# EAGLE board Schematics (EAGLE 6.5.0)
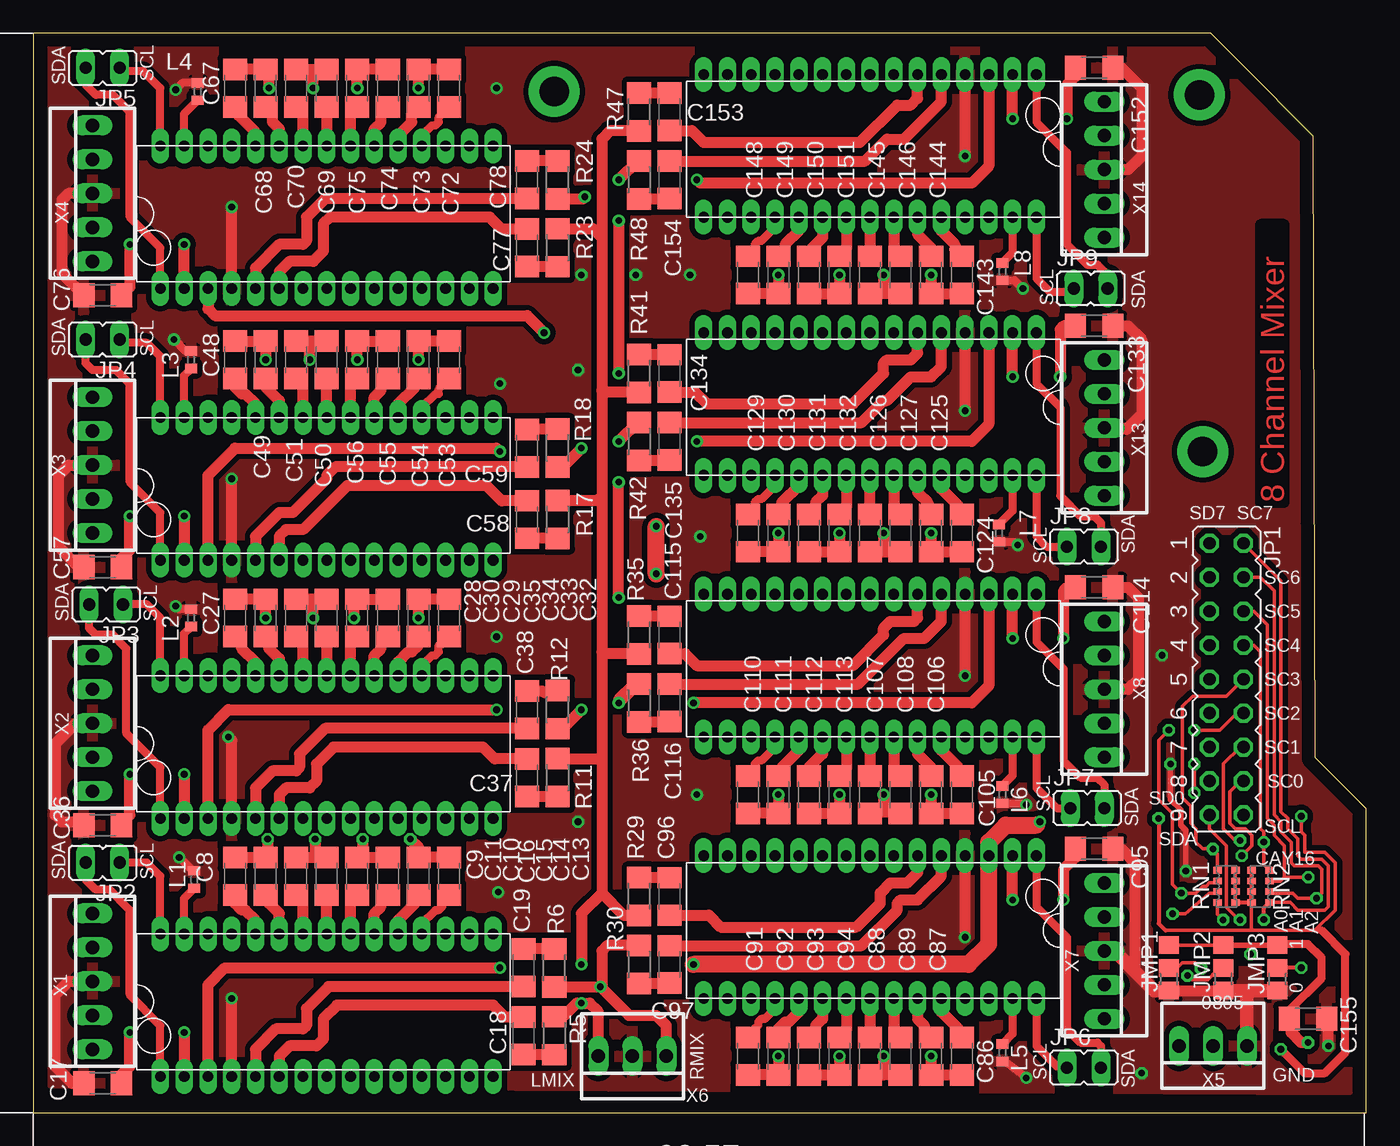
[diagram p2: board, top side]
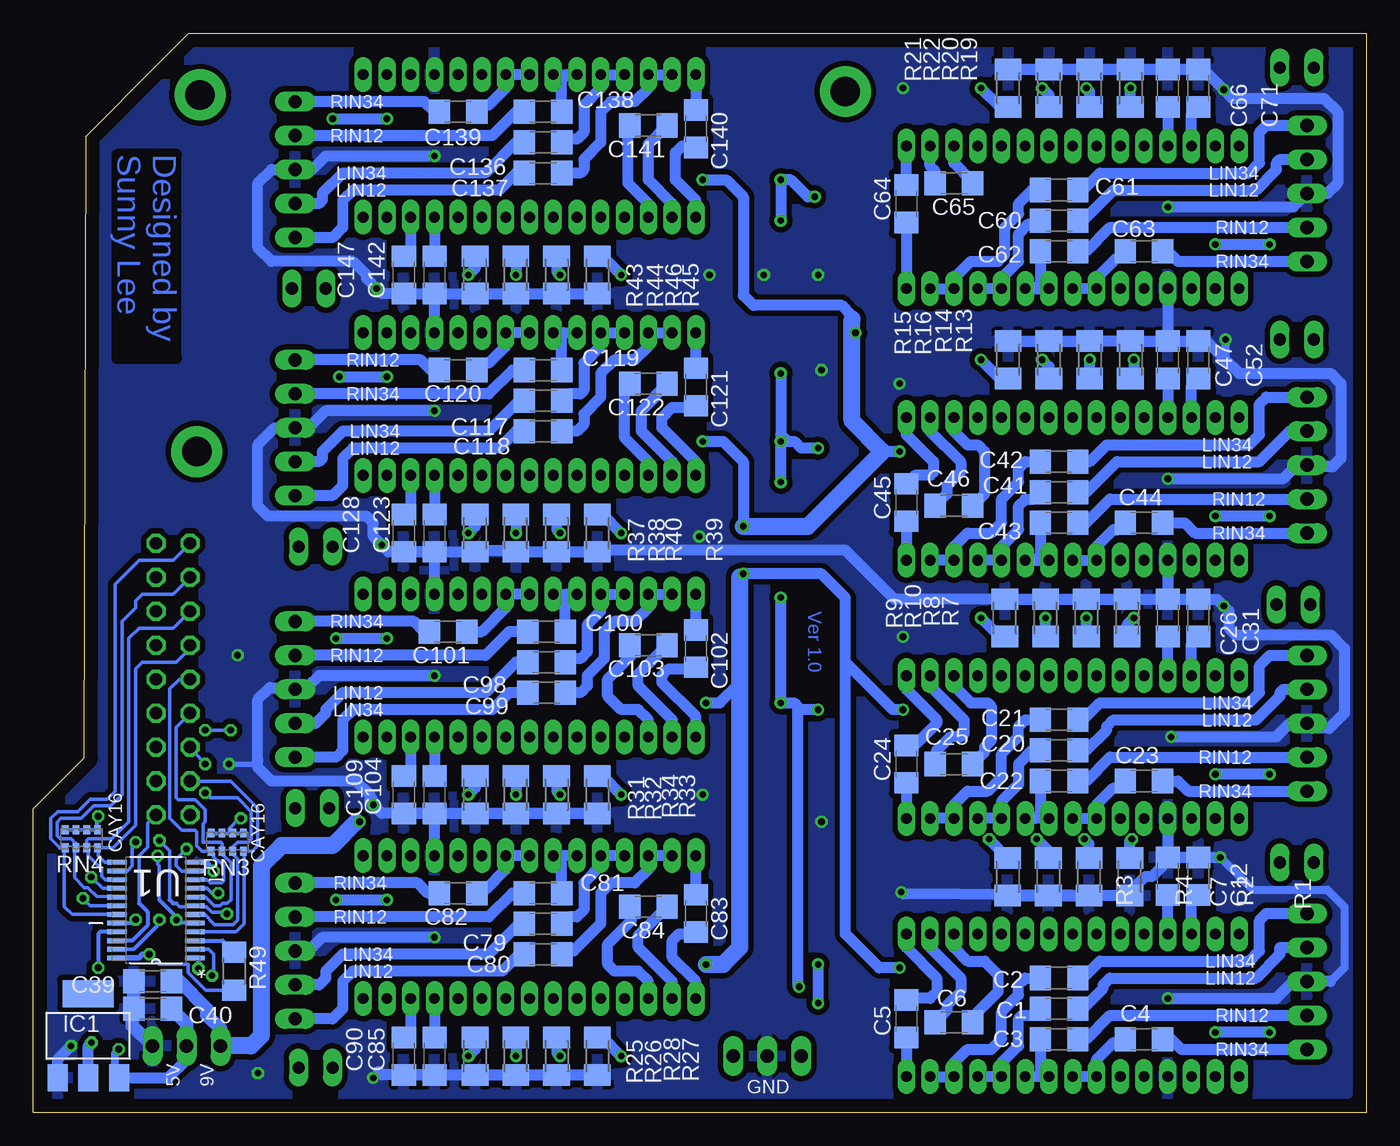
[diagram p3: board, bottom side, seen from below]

Size 99.69 x 80.7 mm. Coordinates in mm from the lower left corner, seen from the top.
Outline: 0,0 99.69,0 99.69,22.73 95.89,26.54 95.76,73.03 90.35,78.44 88.06,80.7 0,80.7 0,0
Copper layers (1*16): Top 0.035mm / dielectric 1.5mm / Bottom 0.035mm
Design rules "default *": minimum track width 10mil, minimum drill 0.4mm, track to track 0.1mm, track to pad 0.1mm, pad to pad 0.1mm, via to via 0.1mm, smd to smd 0.1mm, copper to edge 40mil, drill to drill 8mil, minimum pad ring 10mil, minimum via ring 8mil, stop-mask expansion 4mil, vias tented up to drill 0mil, thermal gap 10mil

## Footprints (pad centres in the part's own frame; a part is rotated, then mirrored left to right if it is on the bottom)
C1206 = smd 1.6 x 1.8: 1 -1.4,0; 2 1.4,0
SOT223 = smd 1.499 x 2.007: 1 -2.261,-3.15; 2 0.025,-3.15; 3 2.311,-3.15 | smd 3.81 x 2.007: 4 0,3.15
B0R-JMP = smd 1.5 x 1.3: 1 0,1.7; 2 0,0; 3 0,-1.7
JP9Q = drill 0.914 octagon: 1 -10.16,-1.27; 2 -10.16,1.27; 3 -7.62,-1.27; 4 -7.62,1.27; 5 -5.08,-1.27; 6 -5.08,1.27; 7 -2.54,-1.27; 8 -2.54,1.27; 9 0,-1.27; 10 0,1.27; 11 2.54,-1.27; 12 2.54,1.27; 13 5.08,-1.27; 14 5.08,1.27; 15 7.62,-1.27; 16 7.62,1.27; 17 10.16,-1.27; 18 10.16,1.27
JP1 = drill 0.914 long: 1 0,-1.27; 2 0,1.27
0402 = smd 0.7 x 0.9: 1 -0.65,0; 2 0.65,0
M1206 = smd 1.6 x 2: 1 -1.4,0; 2 1.4,0
R1206 = smd 1.6 x 1.803: 1 -1.422,0; 2 1.422,0
CAY16 = smd 0.5 x 0.65: 1 -1.2,-0.675; 2 -0.4,-0.675; 3 0.4,-0.675; 4 1.2,-0.675; 5 1.2,0.675; 6 0.4,0.675; 7 -0.4,0.675; 8 -1.2,0.675
SOP65P640X120-24N = smd 1.473 x 0.356: 1 -2.921,3.581; 2 -2.921,2.921; 3 -2.921,2.286; 4 -2.921,1.626; 5 -2.921,0.965; 6 -2.921,0.33; 7 -2.921,-0.33; 8 -2.921,-0.965; 9 -2.921,-1.626; 10 -2.921,-2.286; 11 -2.921,-2.921; 12 -2.921,-3.581; 13 2.921,-3.581; 14 2.921,-2.921; 15 2.921,-2.286; 16 2.921,-1.626; 17 2.921,-0.965; 18 2.921,-0.33; 19 2.921,0.33; 20 2.921,0.965; 21 2.921,1.626; 22 2.921,2.286; 23 2.921,2.921; 24 2.921,3.581
SDIP30 = drill 0.8 long: P$1 1.778,-10.668; P$2 3.556,-10.668; P$3 5.334,-10.668; P$4 7.112,-10.668; P$5 8.89,-10.668; P$6 10.668,-10.668; P$7 12.446,-10.668; P$8 14.224,-10.668; P$9 16.002,-10.668; P$10 17.78,-10.668; P$11 19.558,-10.668; P$12 21.336,-10.668; P$13 23.114,-10.668; P$14 24.892,-10.668; P$15 26.67,-10.668; P$16 26.67,0; P$17 24.892,0; P$18 23.114,0; P$19 21.336,0; P$20 19.558,0; P$21 17.78,0; P$22 16.002,0; P$23 14.224,0; P$24 12.446,0; P$25 10.668,0; P$26 8.89,0; P$27 7.112,0; P$28 5.334,0; P$29 3.556,0; P$30 1.778,0
22-23-2051 = drill 1 long: 1 -5.08,0; 2 -2.54,0; 3 0,0; 4 2.54,0; 5 5.08,0
22-23-2031 = drill 1 long: 1 -2.54,0; 2 0,0; 3 2.54,0

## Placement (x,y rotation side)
C1  0.47u  [C1206]  22.96,7.77 180 bottom
C2  0.47u  [C1206]  22.96,10.06 180 bottom
C3  0.47u  [C1206]  22.96,5.49 180 bottom
C4  0.47u  [C1206]  16.61,5.49 180 bottom
C5  2.2u  [C1206]  34.39,7.01 90 bottom
C6  2.2u  [C1206]  30.84,6.76 0 bottom
C7  5.6n  [C1206]  14.83,17.68 90 bottom
C8  18n  [C1206]  15.09,17.68 90 top
C9  22n  [C1206]  17.37,17.68 90 top
C10  100n  [C1206]  21.95,17.68 90 top
C11  100n  [C1206]  19.66,17.68 90 top
C12  5.6n  [C1206]  12.55,17.68 90 bottom
C13  18n  [C1206]  31.09,17.68 90 top
C14  22n  [C1206]  28.8,17.68 90 top
C15  100n  [C1206]  26.52,17.68 90 top
C16  100n  [C1206]  24.23,17.68 90 top
C17  10u  [C1206]  5.18,2.18 180 top
C18  10u  [C1206]  36.68,5.74 270 top
C19  10u  [C1206]  36.68,10.82 90 top
C20  0.47u  [C1206]  22.96,27.08 180 bottom
C21  0.47u  [C1206]  22.96,29.36 180 bottom
C22  0.47u  [C1206]  22.96,24.79 180 bottom
C23  0.47u  [C1206]  16.61,24.79 180 bottom
C24  2.2u  [C1206]  34.39,26.06 90 bottom
C25  2.2u  [C1206]  30.84,26.06 0 bottom
C26  5.6n  [C1206]  14.83,36.98 90 bottom
C27  18n  [C1206]  15.09,36.98 90 top
C28  22n  [C1206]  17.37,36.98 90 top
C29  100n  [C1206]  21.95,36.98 90 top
C30  100n  [C1206]  19.66,36.98 90 top
C31  5.6n  [C1206]  12.55,36.98 90 bottom
C32  18n  [C1206]  31.09,36.98 90 top
C33  22n  [C1206]  28.8,36.98 90 top
C34  100n  [C1206]  26.52,36.98 90 top
C35  100n  [C1206]  24.23,36.98 90 top
C36  10u  [C1206]  5.18,21.49 180 top
C37  10u  [C1206]  36.93,25.04 270 top
C38  10u  [C1206]  36.93,30.12 90 top
C39  10u  [C1206]  90.78,9.8 180 bottom
C40  10u  [C1206]  90.78,7.77 180 bottom
C41  0.47u  [C1206]  22.96,46.38 180 bottom
C42  0.47u  [C1206]  22.96,48.67 180 bottom
C43  0.47u  [C1206]  22.96,44.09 180 bottom
C44  0.47u  [C1206]  16.61,44.09 180 bottom
C45  2.2u  [C1206]  34.39,45.62 90 bottom
C46  2.2u  [C1206]  30.84,45.36 0 bottom
C47  5.6n  [C1206]  14.83,56.29 90 bottom
C48  18n  [C1206]  15.09,56.29 90 top
C49  22n  [C1206]  17.37,56.29 90 top
C50  100n  [C1206]  21.95,56.29 90 top
C51  100n  [C1206]  19.66,56.29 90 top
C52  5.6n  [C1206]  12.55,56.29 90 bottom
C53  18n  [C1206]  31.09,56.29 90 top
C54  22n  [C1206]  28.8,56.29 90 top
C55  100n  [C1206]  26.52,56.29 90 top
C56  100n  [C1206]  24.23,56.29 90 top
C57  10u  [C1206]  5.18,40.79 180 top
C58  10u  [C1206]  36.93,44.35 270 top
C59  10u  [C1206]  36.93,49.68 90 top
C60  0.47u  [C1206]  22.96,66.7 180 bottom
C61  0.47u  [C1206]  22.96,68.99 180 bottom
C62  0.47u  [C1206]  22.96,64.41 180 bottom
C63  0.47u  [C1206]  16.61,64.41 180 bottom
C64  2.2u  [C1206]  34.39,67.97 90 bottom
C65  2.2u  [C1206]  30.84,69.49 0 bottom
C66  5.6n  [C1206]  14.83,76.61 90 bottom
C67  18n  [C1206]  15.09,76.61 90 top
C68  22n  [C1206]  17.37,76.61 90 top
C69  100n  [C1206]  21.95,76.61 90 top
C70  100n  [C1206]  19.66,76.61 90 top
C71  5.6n  [C1206]  12.55,76.61 90 bottom
C72  18n  [C1206]  31.09,76.61 90 top
C73  22n  [C1206]  28.8,76.61 90 top
C74  100n  [C1206]  26.52,76.61 90 top
C75  100n  [C1206]  24.23,76.61 90 top
C76  10u  [C1206]  5.18,61.11 180 top
C77  10u  [C1206]  36.93,64.67 270 top
C78  10u  [C1206]  36.93,69.75 90 top
C79  0.47u  [C1206]  61.57,14.12 0 bottom
C80  0.47u  [C1206]  61.57,11.84 0 bottom
C81  0.47u  [C1206]  61.57,16.41 0 bottom
C82  0.47u  [C1206]  67.92,16.41 0 bottom
C83  2.2u  [C1206]  50.14,14.88 270 bottom
C84  2.2u  [C1206]  53.7,15.39 180 bottom
C85  5.6n  [C1206]  69.7,4.22 270 bottom
C86  18n  [C1206]  69.44,4.22 270 top
C87  22n  [C1206]  67.16,4.22 270 top
C88  100n  [C1206]  62.59,4.22 270 top
C89  100n  [C1206]  64.87,4.22 270 top
C90  5.6n  [C1206]  71.98,4.22 270 bottom
C91  18n  [C1206]  53.44,4.22 270 top
C92  22n  [C1206]  55.73,4.22 270 top
C93  100n  [C1206]  58.01,4.22 270 top
C94  100n  [C1206]  60.3,4.22 270 top
C95  10u  [C1206]  79.35,19.71 0 top
C96  10u  [C1206]  47.6,16.15 90 top
C97  10u  [C1206]  47.6,11.07 270 top
C98  0.47u  [C1206]  61.32,33.68 0 bottom
C99  0.47u  [C1206]  61.32,31.39 0 bottom
C100  0.47u  [C1206]  61.32,35.97 0 bottom
C101  0.47u  [C1206]  68.68,35.97 0 bottom
C102  2.2u  [C1206]  50.14,34.7 270 bottom
C103  2.2u  [C1206]  53.7,34.95 180 bottom
C104  5.6n  [C1206]  69.7,23.77 270 bottom
C105  18n  [C1206]  69.44,23.77 270 top
C106  22n  [C1206]  67.16,23.77 270 top
C107  100n  [C1206]  62.59,23.77 270 top
C108  100n  [C1206]  64.87,23.77 270 top
C109  5.6n  [C1206]  71.98,23.77 270 bottom
C110  18n  [C1206]  53.44,23.77 270 top
C111  22n  [C1206]  55.73,23.77 270 top
C112  100n  [C1206]  58.01,23.77 270 top
C113  100n  [C1206]  60.3,23.77 270 top
C114  10u  [C1206]  79.35,39.27 0 top
C115  10u  [C1206]  47.6,35.71 90 top
C116  10u  [C1206]  47.6,30.63 270 top
C117  0.47u  [C1206]  61.57,53.24 0 bottom
C118  0.47u  [C1206]  61.57,50.95 0 bottom
C119  0.47u  [C1206]  61.57,55.52 0 bottom
C120  0.47u  [C1206]  67.92,55.52 0 bottom
C121  2.2u  [C1206]  50.14,54.25 270 bottom
C122  2.2u  [C1206]  53.7,54.51 180 bottom
C123  5.6n  [C1206]  69.7,43.33 270 bottom
C124  18n  [C1206]  69.44,43.33 270 top
C125  22n  [C1206]  67.16,43.33 270 top
C126  100n  [C1206]  62.59,43.33 270 top
C127  100n  [C1206]  64.87,43.33 270 top
C128  5.6n  [C1206]  71.98,43.33 270 bottom
C129  18n  [C1206]  53.44,43.33 270 top
C130  22n  [C1206]  55.73,43.33 270 top
C131  100n  [C1206]  58.01,43.33 270 top
C132  100n  [C1206]  60.3,43.33 270 top
C133  10u  [C1206]  79.35,58.83 0 top
C134  10u  [C1206]  47.6,55.27 90 top
C135  10u  [C1206]  47.6,50.19 270 top
C136  0.47u  [C1206]  61.57,72.54 0 bottom
C137  0.47u  [C1206]  61.57,70.26 0 bottom
C138  0.47u  [C1206]  61.57,74.83 0 bottom
C139  0.47u  [C1206]  67.92,74.83 0 bottom
C140  2.2u  [C1206]  50.14,73.56 270 bottom
C141  2.2u  [C1206]  53.7,73.81 180 bottom
C142  5.6n  [C1206]  69.7,62.64 270 bottom
C143  18n  [C1206]  69.44,62.64 270 top
C144  22n  [C1206]  67.16,62.64 270 top
C145  100n  [C1206]  62.59,62.64 270 top
C146  100n  [C1206]  64.87,62.64 270 top
C147  5.6n  [C1206]  71.98,62.64 270 bottom
C148  18n  [C1206]  53.44,62.64 270 top
C149  22n  [C1206]  55.73,62.64 270 top
C150  100n  [C1206]  58.01,62.64 270 top
C151  100n  [C1206]  60.3,62.64 270 top
C152  10u  [C1206]  79.35,78.13 0 top
C153  10u  [C1206]  47.6,74.83 90 top
C154  10u  [C1206]  47.6,69.75 270 top
C155  10u  [C1206]  95.35,7.01 0 top
IC1  REG1117  [SOT223]  95.61,5.74 0 bottom
JMP1  0R-JUMPB  [B0R-JMP]  84.94,10.82 0 top
JMP2  0R-JUMPB  [B0R-JMP]  89,10.82 0 top
JMP3  0R-JUMPB  [B0R-JMP]  93.07,10.82 0 top
JP1  [JP9Q]  89.26,32.41 270 top
JP2  [JP1]  5.18,18.69 90 top
JP3  [JP1]  5.44,38 90 top
JP4  [JP1]  5.18,57.81 90 top
JP5  [JP1]  5.18,78.13 90 top
JP6  [JP1]  78.59,3.35 270 top
JP7  [JP1]  78.84,22.76 270 top
JP8  [JP1]  78.59,42.32 270 top
JP9  [JP1]  79.1,61.62 270 top
L1  BLM15HB121SN1  [0402]  12.04,17.42 90 top
L2  BLM15HB121SN1  [0402]  11.79,36.98 90 top
L3  BLM15HB121SN1  [0402]  11.79,56.29 90 top
L4  BLM15HB121SN1  [0402]  12.29,76.35 90 top
L5  BLM15HB121SN1  [0402]  72.49,4.47 270 top
L6  BLM15HB121SN1  [0402]  72.49,23.77 270 top
L7  BLM15HB121SN1  [0402]  72.24,43.33 270 top
L8  BLM15HB121SN1  [0402]  72.49,62.89 270 top
R1  2.7k  [M1206]  17.68,17.63 270 bottom
R2  5.6k  [M1206]  20.73,17.63 270 bottom
R3  2.7k  [M1206]  26.82,17.63 90 bottom
R4  5.6k  [M1206]  23.77,17.63 90 bottom
R5  10k  [R1206]  38.96,5.74 90 top
R6  10k  [R1206]  38.96,10.82 270 top
R7  2.7k  [M1206]  17.88,36.98 90 bottom
R8  5.6k  [M1206]  20.93,36.98 90 bottom
R9  2.7k  [M1206]  27.03,36.98 270 bottom
R10  5.6k  [M1206]  23.98,36.98 270 bottom
R11  10k  [R1206]  39.22,25.04 90 top
R12  10k  [R1206]  39.22,30.12 270 top
R13  2.7k  [M1206]  17.63,56.29 90 bottom
R14  5.6k  [M1206]  20.68,56.29 90 bottom
R15  2.7k  [M1206]  26.77,56.29 270 bottom
R16  5.6k  [M1206]  23.72,56.29 270 bottom
R17  10k  [R1206]  39.22,44.35 90 top
R18  10k  [R1206]  39.22,49.68 270 top
R19  2.7k  [M1206]  17.63,76.61 90 bottom
R20  5.6k  [M1206]  20.68,76.61 90 bottom
R21  2.7k  [M1206]  26.77,76.61 270 bottom
R22  5.6k  [M1206]  23.72,76.61 270 bottom
R23  10k  [R1206]  39.22,64.67 90 top
R24  10k  [R1206]  39.22,69.75 270 top
R25  2.7k  [M1206]  66.65,4.22 270 bottom
R26  5.6k  [M1206]  63.6,4.22 270 bottom
R27  2.7k  [M1206]  57.51,4.22 90 bottom
R28  5.6k  [M1206]  60.55,4.22 90 bottom
R29  10k  [R1206]  45.31,16.15 270 top
R30  10k  [R1206]  45.31,11.07 90 top
R31  2.7k  [M1206]  66.65,23.77 270 bottom
R32  5.6k  [M1206]  63.6,23.77 270 bottom
R33  2.7k  [M1206]  57.51,23.77 90 bottom
R34  5.6k  [M1206]  60.55,23.77 90 bottom
R35  10k  [R1206]  45.31,35.71 270 top
R36  10k  [R1206]  45.31,30.63 90 top
R37  2.7k  [M1206]  66.65,43.33 270 bottom
R38  5.6k  [M1206]  63.6,43.33 270 bottom
R39  2.7k  [M1206]  57.51,43.33 90 bottom
R40  5.6k  [M1206]  60.55,43.33 90 bottom
R41  10k  [R1206]  45.31,55.27 270 top
R42  10k  [R1206]  45.31,50.19 90 top
R43  2.7k  [M1206]  66.65,62.64 270 bottom
R44  5.6k  [M1206]  63.6,62.64 270 bottom
R45  2.7k  [M1206]  57.51,62.64 90 bottom
R46  5.6k  [M1206]  60.55,62.64 90 bottom
R47  10k  [R1206]  45.31,74.83 270 top
R48  10k  [R1206]  45.31,69.75 90 top
R49  10k  [R1206]  84.68,10.57 90 bottom
RN1  [CAY16]  89.26,16.92 90 top
RN2  [CAY16]  91.8,16.92 270 top
RN3  [CAY16]  85.19,20.22 0 bottom
RN4  [CAY16]  96.11,20.47 0 bottom
U1  PCA9548APWR  [SOP65P640X120-24N]  90.53,15.14 180 bottom
U$1  TDA7439  [SDIP30]  7.72,13.36 0 top
U$2  TDA7439  [SDIP30]  7.72,32.66 0 top
U$3  TDA7439  [SDIP30]  7.72,51.97 0 top
U$4  TDA7439  [SDIP30]  7.72,72.29 0 top
U$5  TDA7439  [SDIP30]  76.81,8.53 180 top
U$6  TDA7439  [SDIP30]  76.81,28.09 180 top
U$7  TDA7439  [SDIP30]  76.81,47.65 180 top
U$8  TDA7439  [SDIP30]  76.81,66.95 180 top
X1  22-23-2051  [22-23-2051]  4.42,9.8 90 top
X2  22-23-2051  [22-23-2051]  4.42,29.11 90 top
X3  22-23-2051  [22-23-2051]  4.42,48.41 90 top
X4  22-23-2051  [22-23-2051]  4.42,68.73 90 top
X5  22-23-2031  [22-23-2031]  88.24,4.98 180 top
X6  22-23-2031  [22-23-2031]  44.81,4.22 180 top
X7  22-23-2051  [22-23-2051]  80.11,12.09 270 top
X8  22-23-2051  [22-23-2051]  80.11,31.65 270 top
X13  22-23-2051  [22-23-2051]  80.11,51.21 270 top
X14  22-23-2051  [22-23-2051]  80.11,70.51 270 top

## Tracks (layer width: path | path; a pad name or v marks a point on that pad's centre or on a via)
5V  (via drill 0.5, 0.5 pad 0.25)
  Top 0.254: RN1.4 RN1.3 RN1.2 RN1.1 | RN2.3 RN2.2 RN2.1 | v94.84,22.15 94.84,20.98 95.1,20.73 95.1,19.46 96.62,19.46 97.38,18.69 97.38,15.14 95.86,13.61 91.29,13.61 | 84.68,13.61 91.29,13.61 | RN2.4 91.12,13.78 91.29,13.61
  Top 0.305: RN1.1 RN2.4 RN2.3 | 95.86,13.61 96.37,13.61 | v84.18,22 84.18,14.12 84.68,13.61
  Top 0.61: v93.32,4.72 95.1,2.95 96.62,2.95 98.15,4.47 98.15,11.84 96.37,13.61
  Bottom 0.254: RN3.5 RN3.6 RN3.7 RN3.8 85.03,20.89 85.06,21.23 84.3,22 v84.18,22
  Bottom 0.305: RN4.8 RN4.7 RN4.6 RN4.5 94.91,21.93 v94.84,22.15 | C40.1 89.38,7.64 88.24,6.5 88.24,3.96 89.76,2.44 92.81,2.44 93.57,3.2 | 93.57,4.47 v93.32,4.72
  Bottom 0.61: 93.57,3.2 93.57,4.47
  Bottom 0.813: IC1.3 89.61,2.59 88.24,3.96 X5.2
  Bottom 1.016: C40.1 88.24,6.63 88.24,6.5 X5.2
9V  (via drill 0.5)
  Top 0.813: U$8.P$3 71.48,70.76 70.21,69.49 49.89,69.49 v49.63,69.75 | U$7.P$3 71.48,51.46 70.21,50.19 v49.63,50.19 | U$3.P$3 13.06,47.65 15.09,49.68 34.65,49.68 v34.9,49.43 | U$4.P$3 13.06,60.1 13.56,59.59 36.93,59.59 v38.2,58.32 | U$2.P$3 13.06,28.6 14.58,30.12 v34.65,30.12 | U$1.P$3 13.06,9.55 14.33,10.82 v34.9,10.82 | U$6.P$3 71.48,31.9 70.21,30.63 v49.38,30.63 | U$5.P$3 71.48,20.22 | 75.03,21.49 v75.29,21.74
  Top 1.27: v46.58,40.28 v46.58,43.84 | v49.38,11.07 69.95,11.07 71.48,12.6 U$5.P$3 | 71.48,20.22 72.75,21.49 75.03,21.49
  Bottom 0.813: v49.63,69.75 47.85,69.75 46.58,68.48 46.58,61.11 45.82,60.35 39.22,60.35 38.46,59.59 38.46,59.33 v38.2,58.32 | v49.63,50.19 48.11,50.19 46.58,48.67 v46.58,43.84 | v34.9,49.43 36.17,49.43 | v34.65,30.12 35.41,30.12 38.96,33.68 | 38.96,33.68 38.96,38.51 40.74,40.28 v46.58,40.28 46.84,40.03 | v34.9,10.82 36.42,10.82 38.96,13.36 38.96,33.68 | v49.38,30.63 48.36,30.63 46.84,32.16 | v75.29,21.74 75.54,21.74
  Bottom 1.016: C39.1 88.75,9.8 86.72,7.77 86.72,7.26 85.7,6.25 X5.3
  Bottom 1.27: 38.46,59.33 38.46,51.71 36.17,49.43 41.76,43.84 v46.58,43.84 | 46.84,40.03 46.84,32.16 46.84,12.34 48.11,11.07 v49.38,11.07 | 75.54,21.74 77.32,19.96 81.13,19.96 82.65,18.44 82.65,5.74 83.41,4.98 X5.3
D1
  Top 0.61: U$1.P$29 11.28,16.01 L1.1
D2
  Top 0.61: U$2.P$29 11.28,35.82 L2.1
D3
  Top 0.61: U$3.P$29 11.28,55.13 L3.1
D4
  Top 0.61: U$4.P$29 11.28,74.69 L4.1
D5
  Top 0.61: U$5.P$29 73.25,5.88 L5.1
D6
  Top 0.61: U$6.P$29 73.25,25.19 L6.1
D7
  Top 0.61: U$7.P$29 73.25,45 L7.1
D8
  Top 0.61: U$8.P$29 73.25,64.3 L8.1
GND  (via drill 0.5)
  Top 0.406: v86.21,18.06 86.21,21.11 85.83,21.49 85.83,22.63 85.06,23.39 v85.06,26.06
  Top 0.61: L1.2 11.9,18.07 v10.9,19.08 | L3.2 11.39,56.94 v10.52,57.81 | L5.2 72.63,3.82 v74.27,2.59 | L6.2 74.16,23.12 v74.27,23.01 | L7.2 73.4,42.68 v73.64,42.44 | L8.2 73.4,62.24 v74.02,61.62 | L4.2 11.17,77 v10.64,76.48 | L2.2 10.88,37.63 v10.64,37.87
  Top 0.813: X4.3 2.64,68.73 2.13,68.22 2.13,62.76 C76.2 | U$4.P$4 v14.83,67.72 | C57.2 3.4,40.79 1.88,42.32 1.88,47.65 2.64,48.41 X3.3 | X2.3 3.15,29.11 1.63,27.58 1.63,22.25 2.13,21.74 3.53,21.74 C36.2 | U$3.P$4 v14.83,47.4 | U$2.P$4 14.83,27.84 v14.58,28.09 | C17.2 2.9,2.18 1.63,3.45 1.63,8.79 2.64,9.8 X1.3 | U$1.P$4 v14.83,8.53 | U$5.P$4 v69.7,13.11 | U$6.P$4 v69.7,32.66 | C114.2 81.89,39.27 82.65,38.51 82.65,32.41 81.89,31.65 X8.3 | U$7.P$4 v69.7,52.48 | C133.2 81.89,58.83 82.91,57.81 82.91,52.22 81.76,51.08 80.75,51.08 80.62,51.21 X13.3 | U$8.P$4 v69.7,71.53 | C152.2 81.38,78.13 82.91,76.61 82.91,71.53 81.89,70.51 X14.3 | JMP1.3 JMP2.3 | C95.2 81.38,19.71 82.4,18.69 82.4,10.57 | v96.88,4.98 96.88,6.89 C155.2
  Top 1.016: JMP1.3 83.84,9.12 82.4,10.57 80.87,12.09 X7.3 | JMP2.3 JMP3.3 91.11,9.12 90.78,8.79 X5.1
  Bottom 0.305: 83.16,26.06 82.91,26.31
  Bottom 0.406: U1.12 86.74,18.72 v86.21,18.06 | v85.06,26.06 83.16,26.06
  Bottom 0.61: C47.2 11.92,57.69 | v10.9,19.08 8.48,16.66 2.9,16.66 1.63,15.39 1.63,10.82 2.64,9.8 | v10.52,57.81 10.52,56.54 10.64,56.41 | v74.27,2.59 74.27,2.69 73.89,3.07 | v74.27,23.01 74.27,23.52 74.52,23.77
  Bottom 0.813: R21.1 R22.1 R20.2 R19.2 C66.2 | C66.2 C71.2 | C66.2 12.17,78.01 v10.64,76.48 10.01,75.84 3.15,75.84 2.13,74.83 2.13,69.49 2.9,68.73 X4.3 5.44,67.72 v14.83,67.72 | R15.1 R16.1 R14.2 R13.2 C47.2 | C47.2 C52.2 11.92,57.69 10.64,56.41 9.5,55.27 2.64,55.27 1.88,54.51 1.88,48.92 2.52,48.28 4.29,48.28 X3.3 5.18,48.41 6.2,47.4 v14.83,47.4 | C26.2 R7.2 R8.2 R10.1 R9.1 35.28,38.38 38.96,42.06 57.38,42.06 R39.1 R40.1 R38.2 63.73,42.06 66.65,42.06 R37.2 C123.2 | C26.2 C31.2 | C26.2 11.15,38.38 v10.64,37.87 10.26,37.49 10.26,36.22 9.75,35.71 2.64,35.71 1.63,34.7 1.63,29.87 2.77,28.73 4.04,28.73 X2.3 5.69,29.11 6.71,28.09 v14.58,28.09 | U$3.P$4 C26.2 | U$4.P$4 C47.2 | R3.1 R4.1 R2.2 R1.2 | C7.2 C12.2 | C7.2 v10.9,19.08 | 2.64,9.8 X1.3 5.44,9.8 6.71,8.53 v14.83,8.53 | C90.2 C85.2 | C85.2 R25.2 R26.2 R28.1 R27.1 | v69.7,13.11 78.08,13.11 79.1,12.09 X7.3 80.87,12.09 | C85.2 73.63,2.82 73.89,3.07 | C109.2 C104.2 | C104.2 R31.2 R32.2 R34.1 R33.1 | v69.7,32.66 78.33,32.66 79.1,31.9 79.86,31.9 X8.3 80.62,31.65 80.75,31.77 82.02,31.77 82.91,30.89 82.91,26.31 82.91,25.81 81.89,24.79 75.54,24.79 74.52,23.77 74.52,23.27 v74.27,23.01 73.63,22.37 C104.2 | U$5.P$4 C104.2 | U$2.P$4 C7.2 | C128.2 C123.2 | v69.7,52.48 77.83,52.48 79.1,51.21 X13.3 81.64,51.21 82.91,49.94 82.91,45.36 82.14,44.6 74.78,44.6 74.27,44.09 74.27,43.08 v73.64,42.44 73.12,41.93 C123.2 | U$6.P$4 C123.2 | 70.21,61.24 C147.2 73.63,61.24 v74.02,61.62 74.78,62.38 74.78,62.64 75.79,63.65 81.89,63.65 82.91,64.67 82.91,69.49 81.89,70.51 X14.3 78.84,70.51 77.83,71.53 v69.7,71.53 | R45.1 R46.1 R44.2 R43.2 C142.2 70.21,61.24
  Bottom 0.813: U$7.P$4 69.7,60.6 69.44,60.86 69.83,60.86 70.21,61.24 | IC1.1 97.87,3.99 v96.88,4.98 | R1.2 34.64,16.36 v34.77,16.48 | R1.2 17.68,16.48 16.51,17.65 16,17.65 15.24,18.41 15.24,18.67 C7.2
  Bottom 1.016: 92.3,7.01 92.18,7.13 C40.2 C39.2 92.18,7.39 92.3,7.26 92.3,7.01 | 92.3,7.01 92.3,6.5 X5.1
  other vias: 49.63,23.77 34.65,76.61 49.12,62.64 34.9,54.51 49.89,43.08 34.65,35.59 82.91,2.95 84.43,34.19 40.74,55.52 41,62.64 45.06,62.64 40.74,21.74
  pour Bottom (isolate 0.406): 1.37,79.91 95.35,79.91 95.35,26.31 98.4,23.27 98.4,1.42 1.37,1.42
  pour Top (isolate 0.406): 1.37,80.16 95.35,80.16 95.35,26.31 98.4,23.27 98.4,1.68 1.37,2.18
LMIX  (via drill 0.5)
  Top 0.813: R5.2 39.73,7.26 40.64,8.18 v41,8.18 41.61,8.18 42.27,7.52 X6.3 | R23.2 41.86,66.09 42.52,65.43 | 42.52,65.43 42.52,54 | 42.52,54 42.52,46.13 | 42.52,46.13 42.52,34.44 | 42.52,34.44 42.52,26.57 | 42.52,26.57 42.52,16.41 | 42.52,16.41 41,14.88 v41,11.07 | R29.2 44.2,14.73 42.52,16.41 | R11.2 42.42,26.47 42.52,26.57 | R35.2 42.67,34.29 42.52,34.44 | R17.2 42.16,45.77 42.52,46.13 | R41.2 42.67,53.85 42.52,54 | R47.2 43.13,73.41 42.52,72.8 42.52,65.43
  Bottom 0.813: v41,11.07 v41,8.18
N$1
  Bottom 0.813: C1.1 21.18,7.77 19.66,9.3 19.66,9.55 19.15,10.06 8.23,10.06 6.45,11.84 6.45,12.34 X1.4
N$2
  Bottom 0.813: U$1.P$12 U$1.P$11 27.28,3.71 26.01,4.98 26.01,7.01 25.76,7.26 24.87,7.26 C1.2
N$3
  Bottom 0.813: C2.1 21.18,10.06 19.91,11.33 8.74,11.33 7.98,12.09 7.98,14.38 7.47,14.88 X1.5
N$4
  Bottom 0.813: U$1.P$14 U$1.P$13 30.84,3.71 29.82,4.72 28.04,4.72 27.28,5.49 27.28,7.52 26.01,8.79 26.01,9.55 25.5,10.06 C2.2
N$5
  Bottom 0.813: C3.1 20.93,5.49 19.15,7.26 X1.2
N$6
  Bottom 0.813: U$1.P$9 24.23,2.69 | 24.23,2.69 U$1.P$10 | C3.2 24.36,2.82 24.23,2.69
N$7
  Bottom 0.813: C4.1 14.58,5.49 13.82,4.72 X1.1
N$8
  Bottom 0.813: U$1.P$8 U$1.P$7 20.17,3.96 18.9,5.23 18.27,5.23 C4.2
N$9
  Bottom 0.813: C5.1 U$1.P$15
N$10
  Bottom 0.813: U$1.P$16 34.39,12.34 32.11,10.06 32.11,9.04 32.61,8.53 34.27,8.53 C5.2
N$11
  Bottom 0.813: U$1.P$17 32.61,12.34 30.33,10.06 30.33,9.04 31.34,8.03 31.34,7.65 C6.1
N$12
  Bottom 0.813: U$1.P$18 30.84,12.34 29.82,11.33 28.55,11.33 27.53,10.31 27.53,9.04 29.06,7.52 29.06,7.13 C6.2
N$13
  Bottom 0.813: U$1.P$27 C7.1
N$14
  Top 0.813: U$1.P$26 16.61,14.38 15.85,15.14 15.6,15.14 15.09,15.65 C8.1
N$15
  Top 0.813: U$1.P$25 18.39,14.88 17.63,15.65 17.63,16.02 C9.1
N$16
  Top 0.813: U$1.P$23 C10.1
N$17
  Top 0.813: U$1.P$24 20.17,15.77 C11.1
N$18
  Bottom 0.813: U$1.P$28 13.06,15.77 C12.1
N$19
  Top 0.61: U$1.P$19 29.06,14.12 30.07,15.14 30.33,15.14 30.58,15.39 30.58,15.77 C13.1
N$20
  Top 0.813: U$1.P$20 27.28,14.38 28.55,15.65 28.55,16.02 C14.1
N$21
  Top 0.813: U$1.P$21 25.5,14.88 26.01,15.39 26.01,15.77 C15.1
N$22
  Top 0.813: U$1.P$22 23.72,15.77 C16.1
N$23  (via drill 0.5)
  Top 0.813: C17.1 6.58,2.82 7.21,3.45 v7.21,5.99 | v11.28,5.99 U$1.P$2
  Bottom 0.813: v7.21,5.99 v11.28,5.99
N$24  (via drill 0.5)
  Top 0.813: C8.2 C9.2 17.53,19.23 v17.53,20.45
  Bottom 0.813: R1.1 17.68,20.3 v17.53,20.45
N$25  (via drill 0.5)
  Top 0.813: C11.2 21.21,19.08 | 21.21,19.08 C10.2 | v21.08,20.45 21.08,19.2 21.21,19.08
  Bottom 0.813: R2.1 20.73,20.09 v21.08,20.45
N$26  (via drill 0.5)
  Top 0.813: C13.2 C14.2 28.8,19.84 v28.19,20.45
  Bottom 0.813: v28.19,20.45 28.19,20.4 R3.2
N$27  (via drill 0.5)
  Top 0.813: C15.2 C16.2 24.64,19.48 v24.64,20.45
  Bottom 0.813: R4.2 23.77,19.58 v24.64,20.45
N$28
  Bottom 0.305: U1.3 85.55,12.85 R49.2
N$29
  Top 0.813: C18.1 35.28,7.14 34.39,8.03 22.71,8.03 21.69,7.01 21.69,5.49 21.18,4.98 19.15,4.98 18.39,4.22 U$1.P$6
N$30
  Top 0.813: C19.1 22.07,9.42 20.42,7.77 20.42,6.5 20.17,6.25 18.14,6.25 16.61,4.72 U$1.P$5
N$31
  Top 0.813: C18.2 38.94,4.34 R5.1
N$32
  Top 0.813: R6.1 36.7,12.24 C19.2
N$33
  Bottom 0.813: U$2.P$12 U$2.P$11 27.28,23.27 26.01,24.54 26.01,26.06 24.99,27.08 C20.2
N$34
  Bottom 0.813: U$2.P$14 U$2.P$13 30.84,23.01 29.82,24.03 28.3,24.03 27.28,25.04 27.28,26.82 26.01,28.09 26.01,28.85 25.5,29.36 C21.2
N$35
  Bottom 0.813: U$2.P$9 24.74,22 | 24.74,22 U$2.P$10 | C22.2 24.36,22.37 24.74,22
N$36
  Bottom 0.813: U$2.P$8 U$2.P$7 20.17,23.01 18.9,24.28 18.52,24.28 C23.2
N$37
  Bottom 0.813: C24.1 U$2.P$15
N$38
  Bottom 0.813: U$2.P$16 34.39,31.65 32.11,29.36 32.11,29.11 33.63,27.58 34.27,27.58 C24.2
N$39
  Bottom 0.813: U$2.P$17 32.61,31.9 30.07,29.36 30.07,28.35 30.33,28.09 31.09,28.09 32.11,27.08 32.11,26.19 C25.1
N$40
  Bottom 0.813: U$2.P$18 30.84,31.9 29.57,30.63 28.3,30.63 28.04,30.38 28.04,27.84 28.55,27.33 28.55,26.95 C25.2
N$41
  Bottom 0.813: U$2.P$27 C26.1
N$42
  Top 0.813: U$2.P$26 16.61,33.68 15.6,34.7 15.6,35.07 C27.1
N$43
  Top 0.813: U$2.P$25 18.39,33.93 17.63,34.7 17.63,35.33 C28.1
N$44
  Top 0.813: C29.1 U$2.P$23
N$45
  Top 0.813: U$2.P$24 20.17,35.07 C30.1
N$46
  Bottom 0.813: U$2.P$28 13.06,35.07 C31.1
N$47
  Top 0.61: U$2.P$19 29.06,33.43 29.82,34.19 30.07,34.19 30.33,34.44 30.33,34.95 30.46,34.95 C32.1
N$48
  Top 0.813: U$2.P$20 27.28,33.68 28.04,34.44 28.3,34.44 28.8,34.95 C33.1
N$49
  Top 0.813: U$2.P$21 25.5,34.19 26.01,34.7 26.01,35.07 C34.1
N$50
  Top 0.813: U$2.P$22 23.72,35.07 C35.1
N$51  (via drill 0.5)
  Top 0.813: C36.1 6.58,21.62 7.21,22.25 v7.21,25.3 | v11.28,25.3 U$2.P$2
  Bottom 0.813: v7.21,25.3 v11.28,25.3
N$52  (via drill 0.5)
  Top 0.813: v17.37,36.98 C28.2 C27.2
  Bottom 0.813: R7.1 17.88,36.47 v17.37,36.98
N$53  (via drill 0.5)
  Top 0.813: C29.2 20.68,38.38 | 20.68,38.38 C30.2 | v20.93,36.98 20.93,38.13 20.68,38.38
  Bottom 0.813: R8.1 v20.93,36.98
N$54  (via drill 0.5)
  Top 0.813: C32.2 29.31,38.38 | 29.31,38.38 C33.2 | v28.8,36.98 28.8,37.87 29.31,38.38
  Bottom 0.813: R9.2 27.4,35.58 v28.8,36.98
N$55  (via drill 0.5)
  Top 0.813: C34.2 C35.2 23.98,38.13 v23.98,36.98
  Bottom 0.813: R10.2 v23.98,36.98
N$56
  Top 0.813: C37.1 34.52,26.44 33.63,27.33 22.45,27.33 21.18,26.06 21.18,24.79 20.68,24.28 18.9,24.28 18.39,23.77 U$2.P$6
N$57
  Top 0.813: C38.1 21.82,28.72 19.91,26.82 19.91,25.81 19.66,25.55 17.88,25.55 16.61,24.28 U$2.P$5
N$58
  Top 0.813: C37.2 39.2,23.64 R11.1
N$59
  Top 0.813: C38.2 38.07,31.52 38.2,31.39 39.07,31.39 R12.1
N$60
  Bottom 0.813: C21.1 21.18,29.36 19.91,30.63 8.74,30.63 7.98,31.39 7.98,33.43 7.21,34.19 X2.5
N$61
  Bottom 0.813: C20.1 20.93,27.08 19.41,28.6 19.41,28.85 18.9,29.36 8.23,29.36 6.45,31.14 6.45,31.39 6.2,31.65 X2.4
N$62
  Bottom 0.813: C22.1 20.93,24.79 19.15,26.57 X2.2
N$63
  Bottom 0.813: C23.1 14.07,24.79 13.31,24.03 X2.1
N$64
  Bottom 0.813: U$3.P$12 U$3.P$11 27.28,42.32 26.01,43.59 26.01,45.36 25.5,45.87 24.87,45.87 C41.2
N$65
  Bottom 0.813: U$3.P$14 U$3.P$13 30.84,42.32 29.82,43.33 28.04,43.33 27.28,44.09 27.28,45.87 26.01,47.14 26.01,48.16 25.5,48.67 C42.2
N$66
  Bottom 0.813: U$3.P$10 24.74,41.3 | 24.74,41.3 U$3.P$9 | C43.2 24.36,41.68 24.74,41.3
N$67
  Bottom 0.813: U$3.P$8 U$3.P$7 20.17,42.32 18.9,43.59 18.52,43.59 C44.2
N$68
  Bottom 0.813: C45.1 U$3.P$15
N$69
  Bottom 0.813: U$3.P$16 34.39,50.7 32.36,48.67 32.36,47.9 32.61,47.65 33.76,47.65 C45.2
N$70
  Bottom 0.813: U$3.P$17 32.61,50.95 30.33,48.67 30.33,47.9 31.34,46.89 31.34,46.26 C46.1
N$71
  Bottom 0.813: U$3.P$18 30.84,50.95 29.82,49.94 29.06,49.94 28.55,49.43 28.55,46.25 C46.2
N$72
  Bottom 0.813: C47.1 U$3.P$27
N$73
  Top 0.813: U$3.P$26 16.61,52.98 15.85,53.75 15.6,53.75 15.09,54.25 C48.1
N$74
  Top 0.813: U$3.P$25 18.39,53.24 17.37,54.25 C49.1
N$75
  Top 0.813: U$3.P$23 C50.1
N$76
  Top 0.813: U$3.P$24 20.17,54.38 C51.1
N$77
  Bottom 0.813: U$3.P$28 13.06,54.38 C52.1
N$78
  Top 0.61: U$3.P$19 29.06,52.73 30.07,53.75 30.33,53.75 30.33,54.12 C53.1
N$79
  Top 0.813: U$3.P$20 27.28,52.98 28.55,54.25 28.55,54.63 C54.1
N$80
  Top 0.813: U$3.P$21 25.5,53.49 26.01,54 26.01,54.38 C55.1
N$81
  Top 0.813: U$3.P$22 23.72,54.38 C56.1
N$82  (via drill 0.5)
  Top 0.813: C57.1 6.58,41.43 7.21,42.06 v7.21,44.6 | v11.28,44.6 U$3.P$2
  Bottom 0.813: v7.21,44.6 v11.28,44.6
N$83  (via drill 0.5)
  Top 0.813: C48.2 C49.2 v17.37,56.29
  Bottom 0.813: v17.37,56.29 17.37,55.14 R13.1
N$84  (via drill 0.5)
  Top 0.813: C50.2 20.93,57.69 | 20.93,57.69 C51.2 | v20.68,56.29 20.68,57.43 20.93,57.69
  Bottom 0.813: R14.1 v20.68,56.29
N$85  (via drill 0.5)
  Top 0.813: C53.2 C54.2 v28.8,56.29
  Bottom 0.813: R15.2 27.4,54.89 v28.8,56.29
N$86  (via drill 0.5)
  Top 0.813: v24.23,56.29 C56.2 C55.2
  Bottom 0.813: R16.2 23.72,55.78 v24.23,56.29
N$87
  Top 0.813: C58.1 35.02,45.75 33.88,46.89 23.47,46.89 20.17,43.59 18.9,43.59 18.39,43.08 U$3.P$6
N$88
  Top 0.813: C59.1 22.58,48.28 21.95,47.65 21.95,47.4 19.41,44.86 18.39,44.86 16.61,43.08 U$3.P$5
N$89
  Top 0.813: R17.1 36.95,42.93 C58.2
N$90
  Top 0.813: R18.1 36.95,51.1 C59.2
N$91
  Bottom 0.813: C43.1 20.93,44.09 19.15,45.87 X3.2
N$92
  Bottom 0.813: C44.1 13.56,44.09 12.8,43.33 X3.1
N$93
  Bottom 0.813: C42.1 20.68,48.67 19.41,49.94 8.74,49.94 7.98,50.7 7.98,52.98 7.47,53.49 X3.5
N$94
  Bottom 0.813: C41.1 20.93,46.38 18.64,48.67 7.98,48.67 5.69,50.95 X3.4
N$95
  Bottom 0.813: U$4.P$12 U$4.P$11 27.28,62.38 26.01,63.65 26.01,65.68 25.25,66.45 24.62,66.45 C60.2
N$96
  Bottom 0.813: U$4.P$14 U$4.P$13 30.84,62.38 29.57,63.65 27.53,63.65 27.03,64.16 27.03,66.19 26.01,67.21 26.01,67.97 24.99,68.99 C61.2
N$97
  Bottom 0.813: U$4.P$10 24.74,61.62 | 24.74,61.62 U$4.P$9 | C62.2 24.36,62 24.74,61.62
N$98
  Bottom 0.813: U$4.P$8 U$4.P$7 20.17,62.38 18.64,63.91 18.52,63.91 C63.2
N$99
  Bottom 0.813: C64.1 U$4.P$15
N$100
  Bottom 0.813: C64.2 U$4.P$16
N$101
  Bottom 0.813: C65.1 32.24,70.39 32.61,70.76 U$4.P$17
N$102
  Bottom 0.813: C65.2 29.44,69.62 30.84,71.02 U$4.P$18
N$103
  Bottom 0.813: C66.1 U$4.P$27
N$104
  Top 0.813: U$4.P$26 16.61,73.3 15.34,74.57 15.34,74.95 C67.1
N$105
  Top 0.813: U$4.P$25 18.39,73.56 17.88,74.07 17.88,74.7 C68.1
N$106
  Top 0.813: C69.1 U$4.P$23
N$107
  Top 0.813: U$4.P$24 20.17,74.7 C70.1
N$108
  Bottom 0.813: U$4.P$28 13.06,74.7 C71.1
N$109
  Top 0.61: U$4.P$19 29.06,73.05 29.82,73.81 30.07,73.81 30.33,74.07 30.33,74.44 C72.1
N$110
  Top 0.813: U$4.P$20 27.28,73.05 28.3,74.07 28.3,74.7 C73.1
N$111
  Top 0.813: U$4.P$21 25.5,73.56 26.01,74.07 26.01,74.7 C74.1
N$112
  Top 0.813: U$4.P$22 23.72,75.34 24.1,75.34 C75.1
N$113  (via drill 0.5)
  Top 0.813: U$4.P$2 v11.28,64.92 | v7.21,64.92 7.21,61.74 C76.1
  Bottom 0.813: v11.28,64.92 v7.21,64.92
N$114  (via drill 0.5)
  Top 0.813: C67.2 C68.2 17.63,77.75 v17.63,76.61
  Bottom 0.813: R19.1 v17.63,76.61
N$115  (via drill 0.5)
  Top 0.813: C70.2 20.68,78.01 | 20.68,78.01 C69.2 | v20.93,76.61 20.93,77.75 20.68,78.01
  Bottom 0.813: R20.1 20.68,76.35 v20.93,76.61
N$116  (via drill 0.5)
  Top 0.813: C72.2 29.31,78.01 | 29.31,78.01 C73.2 | v28.8,76.61 28.8,77.5 29.31,78.01
  Bottom 0.813: R21.2 27.4,75.21 v28.8,76.61
N$117  (via drill 0.5)
  Top 0.813: v24.23,76.61 C75.2 C74.2
  Bottom 0.813: R22.2 23.72,76.1 v24.23,76.61
N$118
  Top 0.813: C77.1 35.02,66.07 34.14,66.95 22.2,66.95 21.69,66.45 21.69,64.41 20.93,63.65 19.15,63.65 18.39,62.89 U$4.P$6
N$119
  Top 0.813: C78.1 21.82,68.35 20.42,66.95 20.42,65.18 20.17,64.92 18.39,64.92 16.61,63.14 U$4.P$5
N$120
  Top 0.813: C77.2 39.2,63.27 R23.1
N$121
  Top 0.813: R24.1 36.95,71.17 C78.2
N$122
  Bottom 0.813: C62.1 20.93,64.41 19.15,66.19 X4.2
N$123
  Bottom 0.813: C63.1 14.83,64.41 14.07,63.65 X4.1
N$124
  Bottom 0.813: C61.1 21.18,68.99 19.91,70.26 8.74,70.26 7.98,71.02 7.98,73.3 7.47,73.81 X4.5
N$125
  Bottom 0.813: C60.1 21.18,66.7 18.9,68.99 8.23,68.99 6.71,70.51 6.71,71.02 6.45,71.27 X4.4
N$126
  Bottom 0.813: U$5.P$12 U$5.P$11 57.25,18.44 58.52,17.17 58.52,15.14 59.03,14.63 59.66,14.63 C79.2
N$127
  Bottom 0.813: U$5.P$14 U$5.P$13 53.7,18.19 54.71,17.17 56.49,17.17 57.25,16.41 57.25,14.12 59.28,12.09 59.92,12.09 C80.2
N$128
  Bottom 0.813: U$5.P$10 60.05,19.2 | 60.05,19.2 U$5.P$9 | C81.2 60.17,19.08 60.05,19.2
N$129
  Bottom 0.813: U$5.P$8 U$5.P$7 64.36,18.19 65.89,16.66 66.27,16.66 C82.2
N$130
  Bottom 0.813: C83.1 U$5.P$15
N$131
  Bottom 0.813: U$5.P$16 50.14,9.8 51.92,11.58 51.92,12.85 51.41,13.36 50.26,13.36 C83.2
N$132
  Bottom 0.813: U$5.P$17 51.92,9.8 54.46,12.34 54.46,13.23 C84.1
N$133
  Bottom 0.813: U$5.P$18 53.7,9.8 54.46,10.57 56.24,10.57 56.74,11.07 56.74,12.6 54.97,14.38 54.97,15.26 C84.2
N$134
  Bottom 0.813: U$5.P$27 C85.1
N$135
  Top 0.813: U$5.P$26 67.92,7.52 69.19,6.25 69.19,5.87 C86.1
N$136
  Top 0.813: U$5.P$25 66.14,7.01 66.65,6.5 66.65,6.12 C87.1
N$137
  Top 0.813: U$5.P$23 C88.1
N$138
  Top 0.813: U$5.P$24 64.36,6.12 C89.1
N$139
  Bottom 0.813: U$5.P$28 71.48,6.12 C90.1
N$140
  Top 0.61: U$5.P$19 55.47,7.77 54.71,7.01 54.46,7.01 54.2,6.76 54.2,6.5 53.95,6.25 53.95,6.12 C91.1
N$141
  Top 0.813: U$5.P$20 57.25,7.52 56.49,6.76 56.24,6.76 55.73,6.25 C92.1
N$142
  Top 0.813: U$5.P$21 59.03,7.01 58.52,6.5 58.52,6.12 C93.1
N$143
  Top 0.813: U$5.P$22 60.81,6.12 C94.1
N$144  (via drill 0.5)
  Top 0.813: C95.1 77.95,19.07 77.06,18.19 v77.06,15.9 | v73.25,15.9 U$5.P$2
  Bottom 0.813: v77.06,15.9 v73.25,15.9
N$145  (via drill 0.5)
  Top 0.813: C86.2 C87.2 v67.16,4.22
  Bottom 0.813: R25.1 66.65,4.72 v67.16,4.22
N$146  (via drill 0.5)
  Top 0.813: C89.2 63.6,2.82 | 63.6,2.82 C88.2 | v63.6,4.22 63.6,2.82
  Bottom 0.813: R26.1 v63.6,4.22
N$147  (via drill 0.5)
  Top 0.813: C91.2 C92.2 v55.73,4.22
  Bottom 0.813: R27.2 57.13,5.62 v55.73,4.22
N$148  (via drill 0.5)
  Top 0.813: C93.2 C94.2 v60.3,4.22
  Bottom 0.813: R28.2 60.55,4.47 v60.3,4.22
N$149
  Top 0.813: C96.1 50.52,14.75 51.41,13.87 61.57,13.87 63.35,15.65 63.35,16.41 64.11,17.17 65.38,17.17 66.14,17.93 U$5.P$6
N$150
  Top 0.813: C97.1 61.95,12.47 64.62,15.14 64.62,15.65 64.87,15.9 66.14,15.9 67.92,17.68 U$5.P$5
N$151
  Top 0.813: C96.2 45.34,17.55 R29.1
N$152
  Top 0.813: R30.1 47.58,9.65 C97.2
N$153
  Bottom 0.813: C81.1 63.86,16.41 65.63,14.63 X7.2
N$154
  Bottom 0.813: C82.1 70.21,16.41 70.97,17.17 X7.1
N$155
  Bottom 0.813: C80.1 63.35,11.84 64.62,10.57 75.79,10.57 76.56,9.8 76.56,7.77 77.32,7.01 X7.5
N$156
  Bottom 0.813: C79.1 63.35,14.12 65.63,11.84 76.56,11.84 77.83,10.57 77.83,10.06 78.33,9.55 X7.4
N$157
  Bottom 0.813: U$6.P$12 U$6.P$11 57.25,37.49 58.27,36.47 58.27,34.44 58.78,33.93 59.66,33.93 C98.2
N$158
  Bottom 0.813: U$6.P$14 U$6.P$13 53.7,37.74 54.71,36.73 56.24,36.73 57,35.97 57,33.93 58.27,32.66 58.27,31.9 58.78,31.39 C99.2
N$159
  Bottom 0.813: U$6.P$9 59.79,38.76 | 59.79,38.76 U$6.P$10 | C100.2 59.92,38.64 59.79,38.76
N$160
  Bottom 0.813: U$6.P$8 U$6.P$7 64.36,37.74 66.14,35.97 C101.2
N$161
  Bottom 0.813: C102.1 U$6.P$15
N$162
  Bottom 0.813: U$6.P$16 50.14,29.62 52.68,32.16 52.68,32.66 52.17,33.17 50.26,33.17 C102.2
N$163
  Bottom 0.813: U$6.P$17 51.92,29.36 54.46,31.9 54.46,32.79 C103.1
N$164
  Bottom 0.813: U$6.P$18 53.7,29.36 54.46,30.12 55.73,30.12 56.74,31.14 56.74,32.41 54.97,34.19 54.97,34.82 C103.2
N$165
  Bottom 0.813: U$6.P$27 C104.1
N$166
  Top 0.813: U$6.P$26 67.92,27.08 69.19,25.81 69.19,25.43 C105.1
N$167
  Top 0.813: U$6.P$25 66.14,26.82 67.16,25.81 C106.1
N$168
  Top 0.813: U$6.P$23 C107.1
N$169
  Top 0.813: U$6.P$24 64.36,25.68 C108.1
N$170
  Bottom 0.813: U$6.P$28 71.48,25.68 C109.1
N$171
  Top 0.61: U$6.P$19 55.47,27.33 54.46,26.31 54.2,26.31 53.95,26.06 53.95,25.55 53.82,25.55 C110.1
N$172
  Top 0.813: U$6.P$20 57.25,27.08 55.98,25.81 55.98,25.43 C111.1
N$173
  Top 0.813: U$6.P$21 59.03,26.82 58.01,25.81 C112.1
N$174
  Top 0.813: U$6.P$22 60.81,25.68 C113.1
N$175  (via drill 0.5)
  Top 0.813: C114.1 77.32,39.27 77.06,39.01 v77.06,35.46 | v73.25,35.46 U$6.P$2
  Bottom 0.813: v77.06,35.46 v73.25,35.46
N$176  (via drill 0.5)
  Top 0.813: v67.16,23.77 C106.2 C105.2
  Bottom 0.813: R31.1 66.65,24.28 v67.16,23.77
N$177  (via drill 0.5)
  Top 0.813: C107.2 62.59,22.5 63.86,22.5 | 63.86,22.5 64.74,22.5 C108.2 | v63.6,23.77 63.6,22.76 63.86,22.5
  Bottom 0.813: R32.1 v63.6,23.77
N$178  (via drill 0.5)
  Top 0.813: C111.2 55.22,22.37 | 55.22,22.37 C110.2 | v55.73,23.77 55.73,22.88 55.22,22.37
  Bottom 0.813: R33.2 57.13,25.17 v55.73,23.77
N$179  (via drill 0.5)
  Top 0.813: C112.2 C113.2 v60.3,23.77
  Bottom 0.813: R34.2 60.55,24.03 v60.3,23.77
N$180
  Top 0.813: C115.1 48.75,34.31 49.63,33.43 61.32,33.43 63.6,35.71 63.6,36.22 64.11,36.73 65.89,36.73 66.14,36.98 U$6.P$6
N$181
  Top 0.813: C116.1 61.7,32.03 65.13,35.46 66.65,35.46 67.92,36.73 U$6.P$5
N$182
  Top 0.813: C115.2 45.34,37.11 R35.1
N$183
  Top 0.813: R36.1 47.58,29.21 C116.2
N$184
  Bottom 0.813: C100.1 64.11,35.97 65.89,34.19 X8.2
N$185
  Bottom 0.813: C101.1 70.46,35.97 71.22,36.73 X8.1
N$186
  Bottom 0.813: C99.1 64.11,31.39 65.38,30.12 75.79,30.12 76.56,29.36 76.56,27.08 77.06,26.57 X8.5
N$187
  Bottom 0.813: C98.1 63.6,33.68 65.89,31.39 76.56,31.39 77.83,30.12 77.83,29.87 78.59,29.11 X8.4
N$188
  Bottom 0.813: U$7.P$12 U$7.P$11 57.25,57.3 58.52,56.03 58.52,54 58.78,53.75 59.66,53.75 C117.2
N$189
  Bottom 0.813: U$7.P$14 U$7.P$13 53.7,57.3 54.71,56.29 56.24,56.29 57.25,55.27 57.25,53.49 58.52,52.22 58.52,51.46 59.03,50.95 C118.2
N$190
  Bottom 0.813: U$7.P$9 60.05,58.32 | 60.05,58.32 U$7.P$10 | C119.2 60.17,58.19 60.05,58.32
N$191
  Bottom 0.813: U$7.P$8 U$7.P$7 64.36,57.3 65.63,56.03 66.01,56.03 C120.2
N$192
  Bottom 0.813: C121.1 U$7.P$15
N$193
  Bottom 0.813: U$7.P$16 50.14,48.67 52.68,51.21 52.68,51.97 51.92,52.73 50.26,52.73 C121.2
N$194
  Bottom 0.813: U$7.P$17 51.92,48.67 54.2,50.95 54.2,52.48 53.19,53.49 53.19,53.62 C122.1
N$195
  Bottom 0.813: U$7.P$18 53.7,48.67 55.47,50.44 55.47,54.13 C122.2
N$196
  Bottom 0.813: U$7.P$27 C123.1
N$197
  Top 0.813: U$7.P$26 67.92,46.63 69.19,45.36 69.19,44.99 C124.1
N$198
  Top 0.813: U$7.P$25 66.14,46.38 66.9,45.62 66.9,44.99 C125.1
N$199
  Top 0.813: C126.1 U$7.P$23
N$200
  Top 0.813: U$7.P$24 64.36,45.24 C127.1
N$201
  Bottom 0.813: U$7.P$28 71.48,45.24 C128.1
N$202
  Top 0.61: U$7.P$19 55.47,46.89 54.46,45.87 54.2,45.87 53.95,45.62 53.95,45.24 C129.1
N$203
  Top 0.813: U$7.P$20 57.25,46.89 55.98,45.62 55.98,44.99 C130.1
N$204
  Top 0.813: U$7.P$21 59.03,46.13 58.52,45.62 58.52,45.24 C131.1
N$205
  Top 0.813: U$7.P$22 60.81,45.24 C132.1
N$206  (via drill 0.5)
  Top 0.813: C133.1 77.06,58.83 76.81,58.57 v76.81,55.02 | v73.25,55.02 U$7.P$2
  Bottom 0.813: v76.81,55.02 v73.25,55.02
N$207  (via drill 0.5)
  Top 0.813: C124.2 C125.2 v67.16,43.33
  Bottom 0.813: R37.1 66.65,43.84 v67.16,43.33
N$208  (via drill 0.5)
  Top 0.813: C126.2 63.35,41.93 | 63.35,41.93 C127.2 | v63.6,43.33 63.6,42.19 63.35,41.93
  Bottom 0.813: R38.1 v63.6,43.33
N$209  (via drill 0.5)
  Top 0.813: C129.2 C130.2 v55.73,43.33
  Bottom 0.813: R39.2 57.13,44.73 v55.73,43.33
N$210  (via drill 0.5)
  Top 0.813: C131.2 C132.2 v60.3,43.33
  Bottom 0.813: R40.2 60.55,43.59 v60.3,43.33
N$211
  Top 0.813: C134.1 49.51,53.87 50.39,52.98 61.32,52.98 63.6,55.27 63.6,56.03 63.86,56.29 65.63,56.29 66.14,56.79 U$7.P$6
N$212
  Top 0.813: C135.1 61.95,51.59 63.6,53.24 63.86,53.24 65.63,55.02 67.16,55.02 67.92,55.78 U$7.P$5
N$213
  Top 0.813: C134.2 45.34,56.67 R41.1
N$214
  Top 0.813: R42.1 47.58,48.77 C135.2
N$215
  Bottom 0.813: C119.1 63.86,55.52 65.63,53.75 X13.2
N$216
  Bottom 0.813: C120.1 69.95,55.52 70.71,56.29 X13.1
N$217
  Bottom 0.813: C118.1 63.6,50.95 64.87,49.68 75.79,49.68 76.56,48.92 76.56,46.89 77.32,46.13 X13.5
N$218
  Bottom 0.813: C117.1 63.35,53.24 65.63,50.95 76.56,50.95 78.08,49.43 78.08,48.92 78.33,48.67 X13.4
N$219
  Bottom 0.813: U$8.P$12 U$8.P$11 57.25,76.61 58.52,75.34 58.52,73.3 59.03,72.8 59.92,72.8 C136.2
N$220
  Bottom 0.813: U$8.P$14 U$8.P$13 53.7,76.61 54.71,75.59 56.49,75.59 57.25,74.83 57.25,72.54 58.52,71.27 58.52,70.51 58.78,70.26 C137.2
N$221
  Bottom 0.813: U$8.P$9 59.79,77.62 | 59.79,77.62 U$8.P$10 | C138.2 60.17,77.24 59.79,77.62
N$222
  Bottom 0.813: U$8.P$8 U$8.P$7 64.36,76.61 65.63,75.34 66.01,75.34 C139.2
N$223
  Bottom 0.813: U$8.P$15 C140.1
N$224
  Bottom 0.813: U$8.P$16 50.14,68.22 51.66,69.75 51.66,71.78 51.16,72.29 50.27,72.29 C140.2
N$225
  Bottom 0.813: 51.92,73.69 C141.1 53.7,72.41 53.7,69.75 51.92,67.97 U$8.P$17
N$226
  Bottom 0.813: U$8.P$18 53.7,67.97 55.22,69.49 55.22,73.69 C141.2
N$227
  Bottom 0.813: U$8.P$27 C142.1
N$228
  Top 0.813: U$8.P$26 67.92,65.94 68.94,64.92 68.94,64.54 C143.1
N$229
  Top 0.813: U$8.P$25 66.14,65.68 67.16,64.67 C144.1
N$230
  Top 0.813: U$8.P$23 C145.1
N$231
  Top 0.813: U$8.P$24 64.36,64.54 C146.1
N$232
  Bottom 0.813: U$8.P$28 71.48,64.54 C147.1
N$233
  Top 0.61: U$8.P$19 55.47,66.19 54.46,65.18 54.2,65.18 53.95,64.92 53.95,64.54 C148.1
N$234
  Top 0.813: U$8.P$20 57.25,65.94 56.24,64.92 56.24,64.54 C149.1
N$235
  Top 0.813: U$8.P$21 59.03,65.43 58.27,64.67 58.27,64.29 C150.1
N$236
  Top 0.813: U$8.P$22 60.81,64.54 C151.1
N$237  (via drill 0.5)
  Top 0.813: C152.1 77.95,77.49 77.32,76.86 v77.32,74.32 | v73.25,74.32 U$8.P$2
  Bottom 0.813: v77.32,74.32 v73.25,74.32
N$238  (via drill 0.5)
  Top 0.813: C143.2 C144.2 v67.16,62.64
  Bottom 0.813: R43.1 66.65,63.14 v67.16,62.64
N$239  (via drill 0.5)
  Top 0.813: C146.2 63.09,61.24 | 63.09,61.24 C145.2 | v63.6,62.64 63.6,61.74 63.09,61.24
  Bottom 0.813: R44.1 v63.6,62.64
N$240  (via drill 0.5)
  Top 0.813: C148.2 C149.2 v55.73,62.64
  Bottom 0.813: R45.2 57.13,64.04 v55.73,62.64
N$241  (via drill 0.5)
  Top 0.813: C150.2 C151.2 v60.3,62.64
  Bottom 0.813: R46.2 60.55,62.89 v60.3,62.64
N$242
  Top 0.813: C153.1 49.25,73.43 50.14,72.54 61.82,72.54 64.62,75.34 65.63,75.34 66.14,75.84 U$8.P$6
N$243
  Top 0.813: C154.1 62.21,71.15 63.86,72.8 65.13,72.8 67.92,75.59 U$8.P$5
N$244
  Top 0.813: C153.2 45.34,76.23 R47.1
N$245
  Top 0.813: R48.1 47.58,68.33 C154.2
N$246
  Bottom 0.813: C138.1 63.6,74.83 65.38,73.05 X14.2
N$247
  Bottom 0.813: C139.1 69.7,74.83 70.46,75.59 X14.1
N$248
  Bottom 0.813: C137.1 63.6,70.26 64.87,68.99 75.79,68.99 76.56,68.22 76.56,66.19 77.32,65.43 X14.5
N$249
  Bottom 0.813: C136.1 63.6,72.54 65.89,70.26 76.56,70.26 78.08,68.73 78.08,68.22 78.33,67.97 X14.4
N$250  (via drill 0.5)
  Top 0.254: RN2.5 94.01,15.72 94.59,15.14 96.62,15.14 96.88,15.39 96.88,18.44 96.37,18.95 94.84,18.95 94.59,19.2 94.59,20.47 93.83,21.23 93.83,22 93.32,22.5 93.32,39.78 JP1.2
  Top 0.305: v92.05,14.43 92.05,15.29 RN2.5
  Bottom 0.305: U1.20 92,14.17 v92.05,14.43
N$251  (via drill 0.5)
  Top 0.254: 92.58,16.41 94.21,16.41 94.59,16.03 v95.99,16.03 96.37,16.41 96.37,18.19 96.11,18.44 94.34,18.44 94.08,18.69 94.08,20.22 93.32,20.98 93.32,21.74 92.81,22.25 92.81,39.01 91.8,40.03 JP1.4
  Top 0.305: 92.58,16.41 RN2.6
  Bottom 0.254: U1.18 95.43,15.47 v95.99,16.03
N$252  (via drill 0.5)
  Top 0.254: v95.38,17.6 93.57,17.6 | 93.57,17.6 93.27,17.3 92.71,17.3 RN2.7 | 93.57,17.6 93.57,19.96 92.81,20.73 92.81,21.49 92.3,22 92.3,36.47 91.29,37.49 JP1.6
  Bottom 0.254: U1.16 94.51,16.76 v95.38,17.6
N$253  (via drill 0.5)
  Top 0.254: RN2.8 92.05,18.54 v92.05,20.22 92.05,20.98 91.8,21.23 91.8,34.44 91.29,34.95 JP1.8
  Bottom 0.254: U1.14 92.69,18.06 92.3,18.44 92.3,19.96 v92.05,20.22
N$254  (via drill 0.5)
  Top 0.254: JP1.10 89.26,31.14 86.72,31.14 85.95,30.38 85.95,23.52 86.59,22.89 86.59,21.61 86.97,21.23 86.97,20.22 87.48,19.71 v88.24,19.71 88.58,19.37 RN1.5
  Bottom 0.254: U1.11 88.62,18.06 89,18.44 89,18.95 v88.24,19.71
N$255  (via drill 0.5)
  Top 0.254: RN1.6 88.47,17.17 87.99,17.17 87.73,16.92 87.48,16.92 86.97,16.41 v85.88,16.41 85.19,17.07 85.19,22.38 84.18,23.39 84.18,27.84 v84.94,28.6 | JP1.12 90.02,29.87 88.75,28.6 v86.84,28.6
  Bottom 0.254: v86.84,28.6 v84.94,28.6 | U1.9 86.69,16.76 86.33,16.41
  Bottom 0.305: 86.33,16.41 v85.88,16.41
N$256  (via drill 0.5)
  Top 0.254: v85.22,14.86 86.18,14.86 87.99,16.41 88.44,16.41 RN1.7 | JP1.14 90.27,27.33 89.03,26.09 89.03,21.21 89.89,20.34 v90.27,20.34
  Bottom 0.254: v90.27,20.34 89.51,19.58 89.51,15.9 | 87.68,15.39 U1.7 | 89,15.65 88.75,15.39 87.68,15.39 | 87.68,15.39 86.78,15.39 86.31,14.97 85.3,14.97
  Bottom 0.305: 89.51,15.9 89.26,15.65 89,15.65 | 85.3,14.97 v85.22,14.86
N$257
  Bottom 0.254: JP1.18 91.16,21.61 91.16,19.84 91.8,19.2 91.8,15.65
  Bottom 0.305: 91.8,15.65 91.16,15.01 91.16,13.99 92.3,12.85 U1.22
N$258
  Top 0.61: U$1.P$30 9.5,17.68 8.48,18.69 JP2.1
N$259  (via drill 0.5)
  Top 0.254: JP1.16 90.27,24.79 89.48,24 89.48,21.64 89.92,21.21 90.68,21.21 91.16,20.73 91.16,19.96 v90.4,19.2 | RN1.8 88.58,14.82 v89,14.4
  Bottom 0.254: v90.4,19.2 90.4,18.57 90.27,18.44 90.27,15.9
  Bottom 0.305: 90.27,15.9 89,14.66 v89,14.4 88.7,14.17 U1.5
N$260
  Top 0.61: U$1.P$1 9.5,6.5 7.21,8.79 7.21,15.14 5.69,16.66 4.67,16.66 3.91,17.42 JP2.2
N$261
  Top 0.61: U$2.P$30 9.5,36.98 8.48,38 JP3.1
N$262
  Top 0.61: U$2.P$1 9.5,25.81 6.96,28.35 6.96,34.7 5.94,35.71 4.67,35.71 4.17,36.22 JP3.2
N$263
  Top 0.61: U$3.P$30 9.5,56.54 8.48,57.56 6.71,57.56 JP4.1
N$264
  Top 0.61: U$3.P$1 9.5,44.86 7.21,47.14 7.21,54.51 6.2,55.52 4.42,55.52 3.91,56.03 JP4.2
N$265
  Top 0.61: U$4.P$30 9.5,76.61 8.23,77.88 6.71,77.88 JP5.1
N$266
  Top 0.61: U$4.P$1 9.5,64.67 7.21,66.95 7.21,74.83 5.94,76.1 4.67,76.1 3.91,76.86 JP5.2
N$267
  Top 0.61: U$5.P$30 75.03,4.98 76.56,3.45 77.06,3.45 JP6.1
N$268
  Top 0.61: U$5.P$1 75.03,15.39 77.32,13.11 77.32,6.25 78.33,5.23 79.6,5.23 79.86,4.98 JP6.2
N$269
  Top 0.61: U$6.P$30 75.03,24.28 76.56,22.76 JP7.1
N$270
  Top 0.61: U$6.P$1 75.03,35.2 77.06,33.17 77.06,26.31 78.33,25.04 79.6,25.04 80.11,24.54 JP7.2
N$271
  Top 0.61: U$7.P$30 75.03,43.08 75.79,42.32 JP8.1
N$272
  Top 0.61: U$7.P$1 75.03,54.51 76.81,52.73 76.81,46.13 78.33,44.6 79.35,44.6 79.86,44.09 JP8.2
N$273
  Top 0.61: U$8.P$30 75.03,62.38 76.05,61.37 77.57,61.37 JP9.1
N$274
  Top 0.61: U$8.P$1 75.03,74.07 77.32,71.78 77.32,64.92 78.84,63.4 79.6,63.4 80.11,62.89 80.11,61.87 JP9.2
N$275  (via drill 0.5)
  Top 0.254: v87.35,10.77 86.92,11.2 85.95,11.2 85.57,10.82 JMP1.2
  Bottom 0.254: U1.1 86.94,11.56 87.35,11.58 87.35,11.33
  Bottom 0.305: 87.35,11.33 v87.35,10.77
N$276  (via drill 0.5)
  Top 0.254: v86.33,10.24 86.67,9.93 87.86,9.93 88.24,10.31
  Top 0.305: 88.24,10.31 88.49,10.31 JMP2.2
  Bottom 0.254: U1.2 86.59,12.22 86.21,11.84 86.21,10.31
  Bottom 0.305: 86.21,10.31 v86.33,10.24
N$277  (via drill 0.5)
  Top 0.305: v94.84,10.82 JMP3.2
  Bottom 0.305: U1.21 94.69,13.51 94.84,13.36 v94.84,10.82
N$278  (via drill 0.5)
  Top 0.254: JMP2.1 JMP1.1
  Top 0.305: C155.1 93.95,7.64 | 93.14,12.6 JMP3.1
  Top 0.406: JMP2.1 90.78,12.52 | 90.78,12.52 JMP3.1 | v91.03,11.84 91.03,12.27 90.78,12.52
  Top 0.61: 93.95,7.64 96.37,10.06 96.37,11.58 95.35,12.6 93.14,12.6
  Top 0.813: v95.35,5.23 94.84,5.23 94.08,5.99 94.08,6.88 C155.1
  Bottom 0.254: R49.1 86.82,9.14 88.11,10.44 88.11,11.07 90.27,11.07 v91.03,11.84
  Bottom 0.406: U1.24 93.8,11.56 93.83,11.58 91.8,11.58 91.54,11.84 v91.03,11.84
  Bottom 0.813: IC1.2 95.58,5 v95.35,5.23
N$279  (via drill 2.2 pad 3.81)
  other vias: 87.48,49.43
N$280  (via drill 2.2 pad 3.81)
  other vias: 87.22,76.1
N$281  (via drill 2.2 pad 3.81)
  other vias: 38.96,76.35
RMIX  (via drill 0.5)
  Top 0.813: R6.2 v42.42,9.4 | v42.42,9.4 44.55,7.26 46.58,7.26 47.35,6.5 X6.1 | R24.2 41.1,68.33 v41.25,68.48 | R30.2 42.93,12.5 42.52,12.09 42.52,9.5 v42.42,9.4 | R12.2 39.57,28.7 v41,30.12 | R36.2 45.31,31.9 44.81,31.9 | 44.81,31.9 43.79,30.89 v43.79,30.63 44.81,31.65 44.81,31.9 | R18.2 39.57,48.26 v41,49.68 | R42.2 45.21,51.61 v43.79,50.19 | R48.2 45.21,71.17 v43.79,69.75 | v43.79,66.7 v43.79,55.27 | v43.79,38.51 v43.79,47.14
  Bottom 0.813: v41.25,68.48 41.76,68.48 43.03,69.75 v43.79,69.75 v43.79,66.7 | 42.52,30.12 42.52,30.38 42.77,30.63 v43.79,30.63 v43.79,38.51 | 42.52,30.12 42.52,9.5 v42.42,9.4 | v41,30.12 42.52,30.12 | v41,49.68 42.27,49.68 42.77,50.19 43.28,50.19 | 43.28,50.19 v43.79,50.19 v43.79,47.14 | v43.79,55.27 43.79,50.7 43.28,50.19
SD0
  Bottom 0.254: U1.4 84.53,13.51 83.92,14.12 83.92,19.47 | RN3.4 83.33,19.54 82.91,19.96 82.91,22.76 84.94,24.79 JP1.15
  Bottom 0.305: 83.92,19.47 RN3.4
SD1  (via drill 0.5)
  Top 0.254: v86.84,26.06 v86.84,23.9
  Bottom 0.254: v86.84,26.06 JP1.13 | v86.84,23.9 86.46,23.52 84.43,23.52 83.39,22.48 83.39,20.42 83.59,20.22 84.43,20.22 84.79,19.86 RN3.3 84.68,19.43 84.68,19.2 84.43,18.95 84.43,14.38 84.76,14.05 86.13,14.05 86.97,14.88 87.53,14.88 U1.6
SD2
  Bottom 0.254: JP1.11 89.03,28.83 89.03,23.55 88.88,23.39 87.61,23.39 86.84,22.63 86.84,21.74 87,21.59 87,20.22 85.7,20.22 85.59,20.11 RN3.2 85.45,19.43 85.45,19.2 84.91,18.67 84.91,15.9 85.19,15.65 85.55,15.65 85.72,15.47 86.16,15.47 86.79,16.1 U1.8
SD3
  Bottom 0.254: U1.10 86.72,17.42 86.49,17.2 85.6,17.2 85.45,17.35 85.45,18.44 85.83,18.82 85.95,18.82 86.21,19.07 86.21,19.36 RN3.1 | 86.46,19.46 86.46,19.47 RN3.1 | RN3.1 87.06,19.54 87.48,19.96 87.48,20.98 87.61,21.11 88.62,21.11 89.48,22 89.48,31.67 88.75,32.41 JP1.9
SD4
  Bottom 0.254: U1.13 94.36,18.72 94.84,19.2 94.84,19.73 | RN4.4 93.74,19.8 92.05,21.49 92.05,33.17 91.54,33.68 89,33.68 88.24,34.44 88.24,34.7 JP1.7
  Bottom 0.305: 94.84,19.73 RN4.4
SD5
  Bottom 0.254: U1.15 94.34,17.42 94.59,17.68 94.59,18.19 95.61,19.2 95.61,19.69 | RN4.3 95.71,20.36 95.61,20.47 93.83,20.47 92.56,21.74 92.56,35.46 91.8,36.22 89.26,36.22 JP1.5
  Bottom 0.305: 95.61,19.69 RN4.3
SD6
  Bottom 0.254: U1.17 94.97,16.15 95.63,16.82 95.89,16.82 96.62,17.55 96.62,19.69 | 96.51,20.11 96.88,20.47 97.69,20.47 97.92,20.7 97.92,21.72 97.64,22 96.11,22 95.2,22.94 93.9,22.94 93.07,23.77 93.07,36.73 92.05,37.74 92.05,38.25 91.54,38.76 89.26,38.76 JP1.3
  Bottom 0.305: 96.62,19.69 RN4.2 96.51,20.11
SD7
  Bottom 0.254: U1.19 96.8,14.81 97.38,15.39 97.38,19.73 | 97.72,19.8 98.4,20.47 98.4,22 97.89,22.5 96.37,22.5 95.43,23.42 94.18,23.42 93.57,24.03 93.57,39.52 91.8,41.3 89.26,41.3 JP1.1
  Bottom 0.305: 97.38,19.73 RN4.1 97.72,19.8
SDA  (via drill 0.5)
  Top 0.254: JP1.17 87.99,21.23 89.26,19.96 89.26,15.34 89.97,14.63 89.99,14.61 89.99,14.4
  Top 0.305: 89.99,14.4 v90.27,14.4
  Bottom 0.254: U1.23 92.18,12.22
  Bottom 0.305: 92.18,12.22 90.27,14.12 v90.27,14.4

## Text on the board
Top: 8 Channel Mixer
Bottom: Designed by / Sunny Lee | Ver 1.0
tPlace: SDA | SCL | SCL | SDA | SDA | SCL | SD7 | SC7 | SDA | SCL | SC6 | SDA | SCL | SC5 | SC4 | SC3 | SC2 | SC1 | SDA | SC0 | SCL | SD0 | SCL | SDA | CAY16 | SDA | SCL | A0 | A1 | A2 | 0805 | 0 1 | SDA | LMIX | RMIX | SCL | GND
bPlace: RIN34 | RIN12 | LIN34 | LIN34 | LIN12 | LIN12 | RIN12 | RIN34 | RIN12 | RIN34 | LIN34 | LIN34 | LIN12 | LIN12 | RIN12 | RIN34 | RIN34 | RIN12 | LIN12 | LIN34 | LIN34 | LIN12 | RIN12 | RIN34 | CAY16 | CAY16 | RIN34 | RIN12 | LIN34 | LIN34 | LIN12 | LIN12 | RIN12 | RIN34 | 9V | 5V | GND
_tNames: C27 | C28 | C30 | C29 | C35 | C34 | C33 | C32 | C36 | C37 | R11 | X2 | C38 | R12 | C8 | C9 | C11 | C10 | C16 | C15 | C14 | C13 | C39 | IC2 | C17 | C18 | R5 | X1 | C19 | R6 | C40 | X10 | X11 | X9 | X12
_bNames: IC1 | R10 | R9 | C31 | C26 | R7 | R8 | C21 | C25 | C24 | C20 | C22 | R4 | R3 | C23 | C12 | C7 | R1 | R2 | C2 | C1 | C6 | C5 | C4 | C3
